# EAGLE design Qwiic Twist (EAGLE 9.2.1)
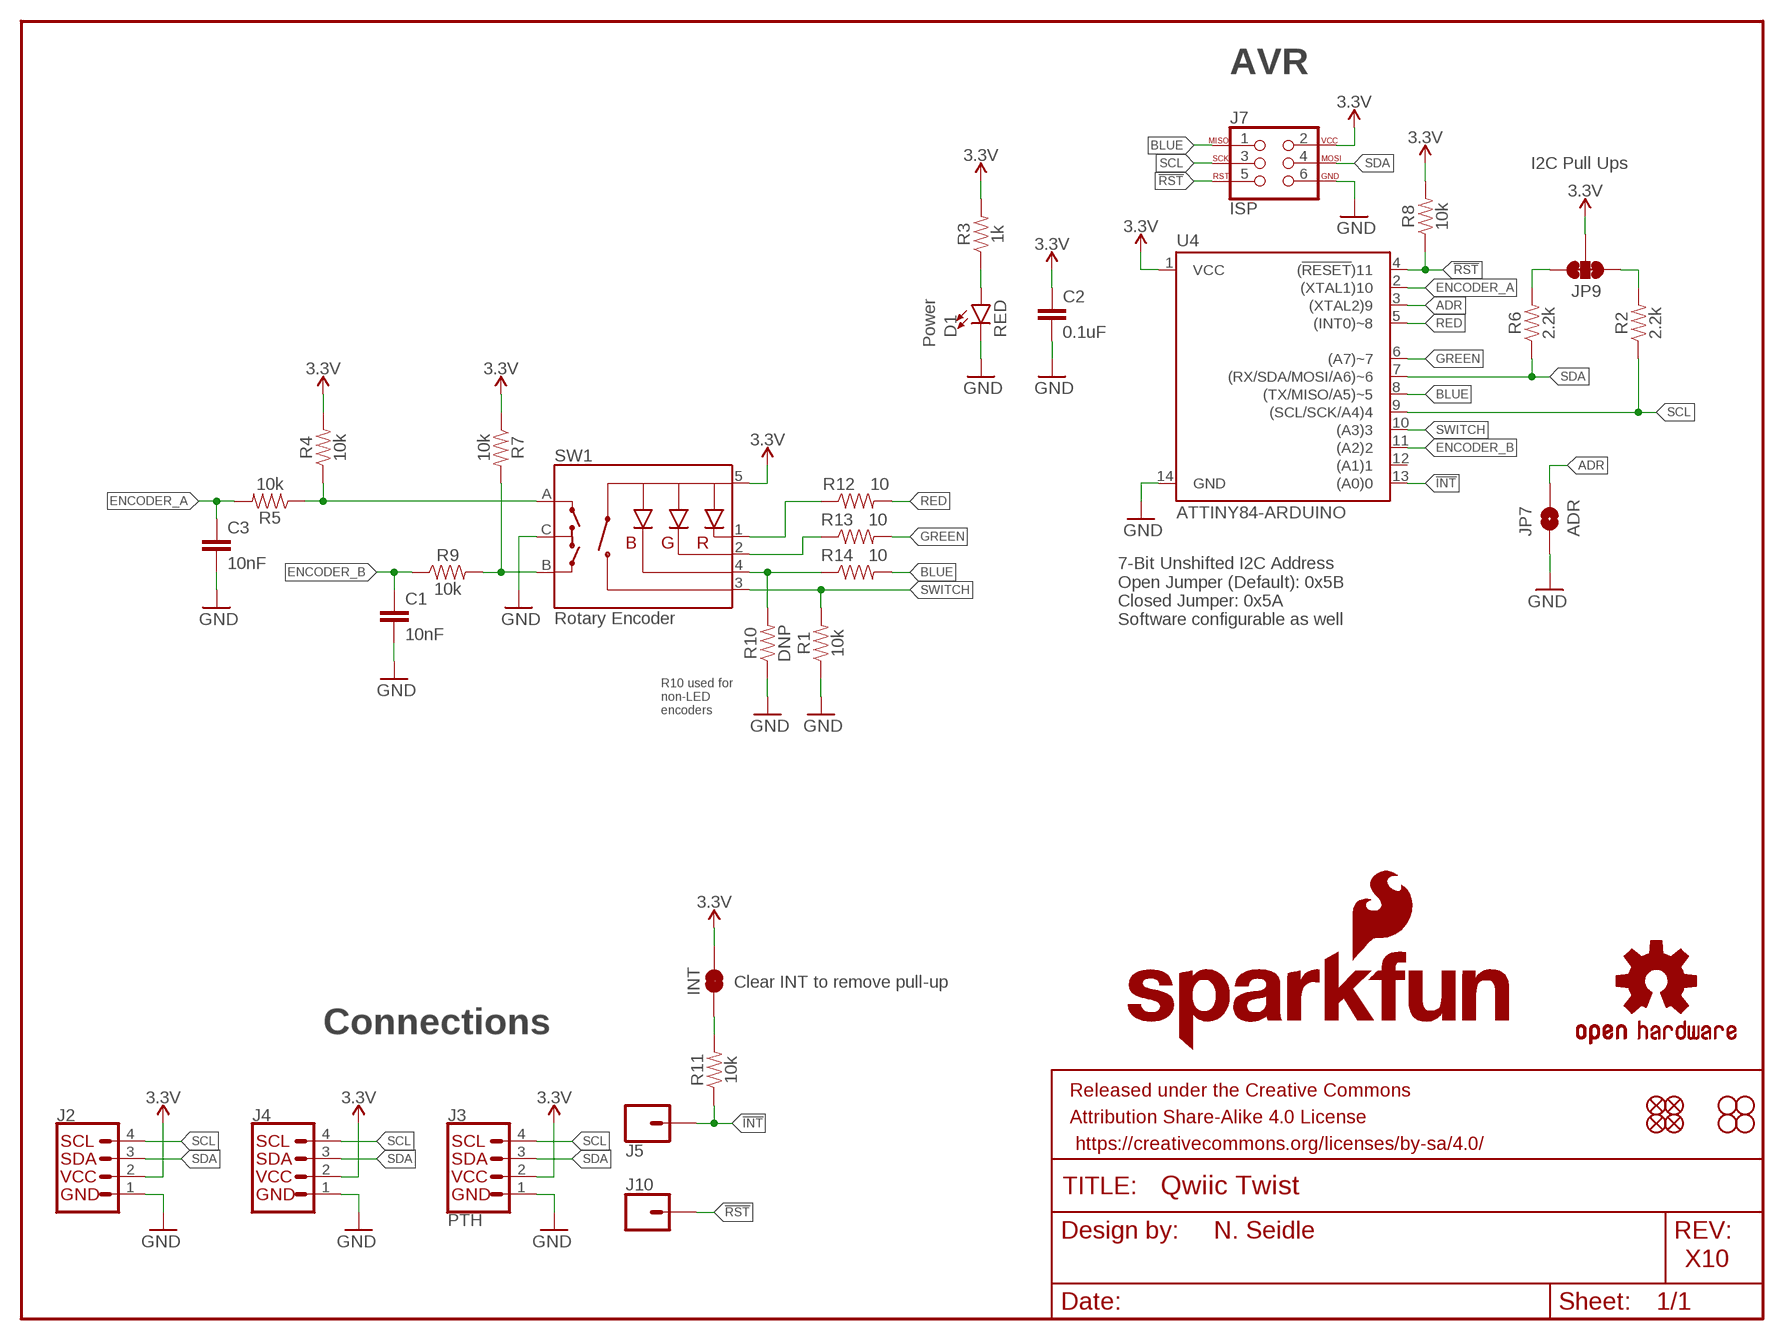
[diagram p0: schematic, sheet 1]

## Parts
C1  10nF  10NF-0603-50V-10%  [0603]
C2  0.1uF  0.1UF-0603-25V-(+80/-20%)  [0603]
C3  10nF  10NF-0603-50V-10%  [0603]
D1  RED  LED-RED0603  [LED-0603]
FRAME1  FRAME-LETTER  [CREATIVE_COMMONS]
INT  JUMPER-SMT_2_NC_TRACE_SILK  [SMT-JUMPER_2_NC_TRACE_SILK]
J2  QWIIC_CONNECTORJS-1MM  [1X04_1MM_RA]
J3  PTH  I2C_STANDARD_NO_SILK  [1X04_NO_SILK]
J4  QWIIC_CONNECTORJS-1MM  [1X04_1MM_RA]
J5  CONN_01PTH_NO_SILK_YES_STOP  [1X01_NO_SILK]
J7  ISP  AVR_SPI_PROG_3X2TESTPOINTS  [2X3_TEST_POINTS]
J10  CONN_01PTH_NO_SILK_YES_STOP  [1X01_NO_SILK]
JP1  FIDUCIALUFIDUCIAL  [MICRO-FIDUCIAL]
JP2  FIDUCIALUFIDUCIAL  [MICRO-FIDUCIAL]
JP3  STAND-OFF  [STAND-OFF]
JP4  STAND-OFF  [STAND-OFF]
JP5  FIDUCIALUFIDUCIAL  [MICRO-FIDUCIAL]
JP6  FIDUCIALUFIDUCIAL  [MICRO-FIDUCIAL]
JP7  ADR  JUMPER-SMT_2_NO_SILK  [SMT-JUMPER_2_NO_SILK]
JP9  JUMPER-SMT_3_2-NC_TRACE_SILK  [SMT-JUMPER_3_2-NC_TRACE_SILK]
JP11  STAND-OFF  [STAND-OFF]
JP13  STAND-OFF  [STAND-OFF]
LOGO1  OSHW-LOGOMINI  [OSHW-LOGO-MINI]
LOGO2  SFE_LOGO_NAME_FLAME.1_INCH  [SFE_LOGO_NAME_FLAME_.1]
LOGO3  SFE_LOGO_FLAME.1EXP  [SFE_LOGO_FLAME_COPPER_EXPOSED_.1]
R1  10k  10KOHM-0603-1/10W-1%  [0603]
R2  2.2k  2.2KOHM-0603-1/10W-1%  [0603]
R3  1k  1KOHM-0603-1/10W-1%  [0603]
R4  10k  10KOHM-0603-1/10W-1%  [0603]
R5  10k  10KOHM-0603-1/10W-1%  [0603]
R6  2.2k  2.2KOHM-0603-1/10W-1%  [0603]
R7  10k  10KOHM-0603-1/10W-1%  [0603]
R8  10k  10KOHM-0603-1/10W-1%  [0603]
R9  10k  10KOHM-0603-1/10W-1%  [0603]
R10  DNP  10KOHM-0603-1/10W-1%  [0603]
R11  10k  10KOHM-0603-1/10W-1%  [0603]
R12  10  10OHM-0603-1/10W-1%  [0603]
R13  10  10OHM-0603-1/10W-1%  [0603]
R14  10  10OHM-0603-1/10W-1%  [0603]
SW1  Rotary Encoder  ENCODER-RGB-SWITCHKIT  [ENCODER_LED_3_KIT]
U4  ATTINY84-ARDUINO  [SO14]

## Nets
3.3V: C2.1 INT.2 J2.2 J3.2(VCC) J4.2 J7.2 JP9.2 R3.2 R4.2 R7.1 R8.2 SW1.5(+) U4.1(VCC)
!INT: J5.1 R11.1 U4.13((A0)0)
!RST: J7.5 J10.1 R8.1 U4.4((!RESET!)11)
A: R4.1 R5.1 SW1.A
ADR: JP7.2 U4.3((XTAL2)9)
B: R7.2 R9.2 SW1.B
BLUE: J7.1 R14.2 U4.8((TX/MISO/A5)~5)
BLUE_RAW: R10.2 R14.1 SW1.4(-B)
ENCODER_A: C3.1 R5.2 U4.2((XTAL1)10)
ENCODER_B: C1.1 R9.1 U4.11((A2)2)
GND: C1.2 C2.2 C3.2 D1.C J2.1 J3.1(GND) J4.1 J7.6 JP7.1 R1.1 R10.1 SW1.C U4.14(GND)
GREEN: R13.2 U4.6((A7)~7)
GREEN_RAW: R13.1 SW1.2(-G)
INT_R: INT.1 R11.2
N$3: D1.A R3.1
RED: R12.2 U4.5((INT0)~8)
RED_RAW: R12.1 SW1.1(-R)
SCL: J2.4 J3.4(SCL) J4.4 J7.3 R2.1 U4.9((SCL/SCK/A4)4)
SCL_PU1: JP9.1 R2.2
SDA: J2.3 J3.3(SDA) J4.3 J7.4 R6.1 U4.7((RX/SDA/MOSI/A6)~6)
SDA_PU1: JP9.3 R6.2
SWITCH: R1.2 SW1.3(SW) U4.10((A3)3)
Unconnected: U4.12((A1)1)

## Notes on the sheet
- AVR
- I2C Pull Ups
- Power
- 7-Bit Unshifted I2C Address
  Open Jumper (Default): 0x5B
  Closed Jumper: 0x5A
  Software configurable as well
- R10 used for 
  non-LED 
  encoders
- Clear INT to remove pull-up
- Connections
- N. Seidle
- X10

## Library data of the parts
C1 C3 = SparkFun-Capacitors:10NF: 0.01uF/10nF/10,000pF ceramic capacitors; PROD_ID: CAP-00867
C2 = SparkFun-Capacitors:0.1UF: 0.1µF ceramic capacitors; PROD_ID: CAP-00810
D1 = SparkFun-LED:LED-RED: Red SMD LED; PROD_ID: DIO-00819
FRAME1 = SparkFun-Aesthetics:FRAME-LETTER: Schematic Frame - Letter
INT = SparkFun-Jumpers:JUMPER-SMT_2_NC_TRACE: Normally closed trace jumper
J2 J4 = SparkFun-Connectors:QWIIC_CONNECTOR: SparkFun I2C Standard Qwiic Connector An SMD 1mm pitch JST connector makes it easy and quick (get it? Qwiic?) to connect I2C devices to each other. The Qwiic system enables fast and solderless connection between popular platforms and various sensors and actuators. We carry 200mm, 100mm, 50mm, and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; PROD_ID: CONN-13694
J3 = SparkX:I2C_STANDARD: SparkFun I2C Standard Pinout Header SparkFun has standardized on a pinout for all I2C based sensor breakouts. This pinout allows I2C boards to be plugged directly into the headers on Arduino Uno compatible boards, and to be daisy chained easily. Example SparkFun Products: SparkFun Atmospheric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
J5 J10 = SparkFun-Connectors:CONN_01: Single connection point. Often used as Generic Header-pin footprint for 0.1 inch spaced/style header connections
J7 = SparkFun-Connectors:AVR_SPI_PROG_3X2: AVR ISP 6 Pin This is the reduced ISP connector for AVR programming. Common on Arduino. This footprint will take up less PCB space and can be used with a 10-pin to 6-pin adapter such as SKU: BOB-08508 **Special note about "TEST_POINT" package. The stop mask is on the top side, so if you want your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
JP1 JP2 JP5 JP6 = SparkFun:FIDUCIAL: Fiducial Alignment Points
JP3 JP4 JP11 JP13 = SparkFun:STAND-OFF: Stand Off
JP7 = SparkFun-Jumpers:JUMPER-SMT_2_NO: Normally open jumper
JP9 = SparkFun-Jumpers:JUMPER-SMT_3_2-NC_TRACE: Normally closed trace jumper (2 of 2 connections) This jumper has a trace between all three pads so they are normally closed (NC). Use a razor knife to open the connection(s). For best results follow the IPC guidelines for cutting traces: Cutout at least 0.063 mm (0.005 in). Remove all loose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
LOGO1 = SparkFun-Aesthetics:OSHW-LOGO: Open-Source Hardware (OSHW) Logo
LOGO2 = SparkFun-Aesthetics:SFE_LOGO_NAME_FLAME: SparkFun Font Logo w/ Flame
LOGO3 = SparkFun-Aesthetics:SFE_LOGO_FLAME: SparkFun Flame Logo
R1 R4 R5 R7-R9 R11 = SparkFun-Resistors:10KOHM: 10kΩ resistor; PROD_ID: RES-00824
R2 R6 = SparkFun-Resistors:2.2KOHM: 2.2kΩ resistor; PROD_ID: RES-08272
R3 = SparkFun-Resistors:1KOHM: 1kΩ resistor; PROD_ID: RES-07856
R10 = SparkFun-Resistors:10KOHM: 10kΩ resistor; PROD_ID: RES-00824; VALUE: 10k
R12-R14 = SparkFun-Resistors:10OHM: 10Ω resistor; PROD_ID: RES-12581
SW1 = SparkFun-Switches:ENCODER-RGB-SWITCH: Illuminated Rotary Encoder w/ RGB LED and select switch Encoders rotate similarly to potentiometers, but they’re different from potentiometers in that an encoder has full rotation without limits. They output gray code so that you can tell how much and in which direction the encoder has been turned.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; PROD_ID: RES-10859; SF_SKU: COM-10982
U4 = SparkFun-IC-Microcontroller:ATTINY84-ARDUINO; PROD_ID: IC-14155

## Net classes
1 3.3V: width 0.152 mm

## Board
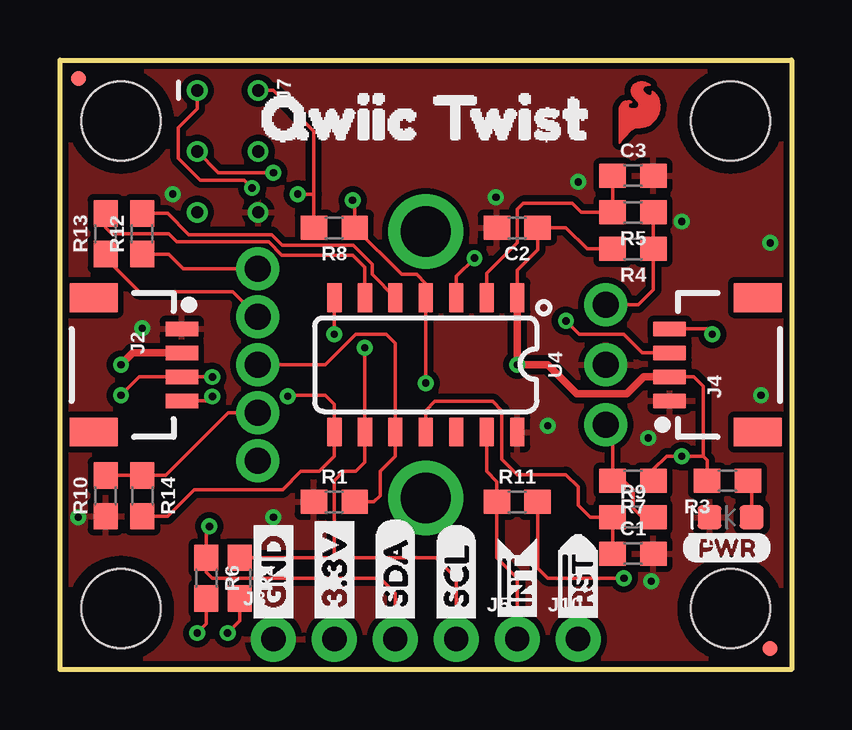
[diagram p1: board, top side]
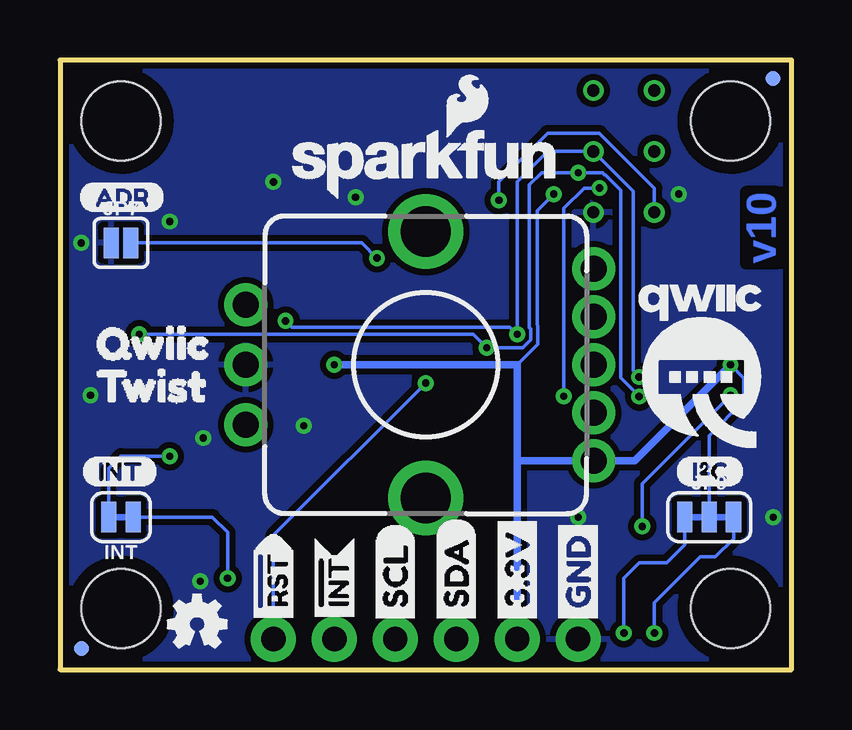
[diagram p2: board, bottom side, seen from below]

Size 30.48 x 25.4 mm. Coordinates in mm from the lower left corner, seen from the top.
Outline: 0,0 0,25.4 30.48,25.4 30.48,0 0,0
Copper layers (1*16): Top 0.035mm / dielectric 1.5mm / Bottom 0.035mm
Design rules "SparkFun-2-layer-PCBWay-LIMIT *": minimum track width 6mil, minimum drill 0.3mm, track to track 6mil, track to pad 6mil, pad to pad 6mil, via to via 6mil, smd to smd 6mil, copper to edge 6mil, drill to drill 6mil, minimum pad ring 7mil, minimum via ring 7mil, stop-mask expansion 4mil, vias tented up to drill 25mil, thermal gap 10mil

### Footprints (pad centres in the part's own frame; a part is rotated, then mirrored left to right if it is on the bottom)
0603 = smd 1.1 x 1: 1 -0.85,0; 2 0.85,0
LED-0603 = smd 1 x 1: A -0.877,0; C 0.877,0
SMT-JUMPER_2_NC_TRACE_SILK = smd 0.635 x 1.27: 1 -0.508,0; 2 0.508,0
1X04_1MM_RA = smd 0.6 x 1.35: 1 -1.5,0; 2 -0.5,0; 3 0.5,0; 4 1.5,0 | smd 1.2 x 2: NC1 2.8,-3.675; NC2 -2.8,-3.675
1X04_NO_SILK = drill 1.016 pad 1.88: 1 0,0; 2 2.54,0; 3 5.08,0; 4 7.62,0
1X01_NO_SILK = drill 1.016 pad 1.88: 1 0,0
2X3_TEST_POINTS = drill 0.508: 1 -2.54,-1.27; 2 -2.54,1.27; 3 0,-1.27; 4 0,1.27; 5 2.54,-1.27; 6 2.54,1.27
MICRO-FIDUCIAL = smd 0.635 x 0.635: 1 0,0
STAND-OFF = hole 3.302: 0,0
SMT-JUMPER_2_NO_SILK = smd 0.635 x 1.27: 1 -0.406,0; 2 0.406,0
SMT-JUMPER_3_2-NC_TRACE_SILK = smd 0.635 x 1.27: 1 -1.016,0; 2 0,0; 3 1.016,0
ENCODER_LED_3_KIT = drill 1.1 pad 1.778: 1 -4,7; 2 -2,7; 3 0,7; 4 2,7; 5 4,7 | drill 1.1 pad 1.8: A -2.5,-7.5; B 2.5,-7.5; C 0,-7.5 | drill 2.1: M1 -5.55,0; M2 5.55,0
SO14 = smd 0.6 x 1.2: 1 -3.175,-2.8; 2 -1.905,-2.8; 3 -0.635,-2.8; 4 0.635,-2.8; 5 1.905,-2.8; 6 3.175,-2.8; 7 4.445,-2.8; 8 4.445,2.8; 9 3.175,2.8; 10 1.905,2.8; 11 0.635,2.8; 12 -0.635,2.8; 13 -1.905,2.8; 14 -3.175,2.8

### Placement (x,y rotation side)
C1  23.88,4.83 0 top
C2  19.05,18.41 180 top
C3  23.88,20.57 0 top
D1  27.94,6.35 180 top
FRAME1  not placed on the board
INT  27.94,6.35 180 bottom
J2  5.08,12.7 270 top
J3  8.89,1.27 0 top
J4  25.4,12.7 90 top
J5  19.05,1.27 0 top
J7  6.99,21.59 270 top
J10  21.59,1.27 0 top
JP1  0.76,24.64 0 bottom
JP2  29.59,0.89 0 top
JP3  2.54,22.86 0 top
JP4  27.94,22.86 0 top
JP5  29.59,0.89 0 bottom
JP6  0.76,24.64 0 top
JP7  27.94,17.78 0 bottom
JP9  3.43,6.35 0 bottom
JP11  2.54,2.54 0 top
JP13  27.94,2.54 0 top
LOGO1  24.77,1.91 0 bottom
LOGO2  15.24,21.08 0 bottom
LOGO3  24.13,23.24 0 top
R1  11.43,6.99 0 top
R2  7.49,3.81 270 top
R3  27.81,7.87 180 top
R4  23.88,17.53 180 top
R5  23.88,19.05 180 top
R6  6.1,3.81 270 top
R7  23.88,7.87 180 top
R8  11.43,18.41 180 top
R9  23.88,6.35 0 top
R10  1.91,7.24 90 top
R11  19.05,6.99 0 top
R12  3.43,18.16 90 top
R13  1.91,18.16 90 top
R14  3.43,7.24 270 top
SW1  15.24,12.7 270 bottom
U4  15.88,12.7 180 top
U$1  [QWIIC1]  30.1,13.59 0 bottom
U$2  [INT0]  29.59,8.26 0 bottom
U$3  [GND1]  8.89,1.65 90 bottom
U$4  [3#3V2]  11.43,1.65 90 bottom
U$5  [SDA8]  13.97,1.65 90 bottom
U$6  [SCL9]  16.51,1.65 90 bottom
U$7  [RST#-[>]  21.59,1.52 90 top
U$8  [I_SUPER2_C-()-03]  4.83,8.26 0 bottom
U$9  [INT#-[<]  19.05,1.52 90 top
U$11  [INT#-[<]  19.05,1.52 90 bottom
U$12  [TWIST2]  30.1,11.81 0 bottom
U$14  [QWIIC_TWIST1]  6.73,22.99 0 top
U$16  [RST#-[>]  21.59,1.52 90 bottom
U$17  [PWR-()-03]  25.91,5.08 0 top
U$18  [ADR-()-03]  29.72,19.68 0 bottom
U$21  [3#3V2]  11.43,1.65 90 top
U$22  [GND1]  8.89,1.65 90 top
U$26  [SCL9]  16.51,1.65 90 top
U$27  [SDA8]  13.97,1.65 90 top
U$47  [QWIIC-LOGO-MEDIUM]  3.81,12.7 0 bottom

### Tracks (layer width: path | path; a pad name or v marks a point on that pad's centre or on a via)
3.3V  (via drill 0.3)
  Top 0.152: U4.1 19.05,16.64 19.9,17.49 C2.1 21.08,18.41 21.97,17.53 R4.2 | J7.2 8.89,24.13 10.58,22.44 10.58,19.81 | R8.2 10.58,19.81 | R7.1 24.73,8.34 25.27,8.89 v25.91,8.89 26.8,8.89 | J4.2 26.41,12.2 26.8,11.81 26.8,8.89 | v9.91,19.81 10.58,19.81 | R3.2 26.96,8.72 26.8,8.89
  Top 0.305: J4.2 24.32,12.2 23.62,11.49 21.52,11.49 20.32,12.7 v19.05,12.7 U4.1 | J2.2 3.04,13.2 v2.54,12.7
  Bottom 0.152: v9.91,19.81 10.6,19.11 10.6,14.37 10.57,14.33 10.57,13.56 11.43,12.7 | INT.2 28.45,8.38 27.94,8.89 v25.91,8.89 | JP9.2 3.43,9.75 1.98,11.2 1.98,12.14 v2.54,12.7
  Bottom 0.305: 8.38,8.7 SW1.5 | SW1.5 6.54,8.7 v2.54,12.7 | J3.2 11.43,8.64 | 11.43,8.64 11.37,8.7 SW1.5 | v19.05,12.7 11.43,12.7 11.43,8.64
!INT
  Top 0.152: J5.1 19.05,3.81 18.2,4.66 R11.1 18.2,7.83 17.78,8.26 U4.13
!RST  (via drill 0.3)
  Top 0.152: v12.19,19.56 12.28,19.47 R8.1 14.23,16.46 14.86,16.46 15.24,16.08 U4.4 v15.24,11.94
  Bottom 0.152: v12.19,19.56 12.19,20.32 10.16,22.35 8,22.35 5.71,20.07 J7.5 | J10.1 21.59,5.59 v15.24,11.94
A
  Top 0.152: R5.1 R4.1 24.73,15.84 24.09,15.2 SW1.A
ADR  (via drill 0.3)
  Top 0.152: U4.3 16.51,16.38 v17.27,17.14
  Bottom 0.152: JP7.2 17.91,17.78 v17.27,17.14
B
  Top 0.152: R9.2 24.26,6.35 23.88,6.73 23.88,7.49 23.5,7.87 R7.2 23.03,9.91 SW1.B
BLUE  (via drill 0.3)
  Top 0.152: v9.49,11.39 9.53,11.43 11.05,11.43 11.43,11.05 U4.8 11.43,8.89 10.79,8.26 10.03,8.26 9.27,7.49 5.59,7.49 4.48,6.39 R14.2 | v8,20.07 7.67,20.4 5.85,20.4 4.93,21.32 4.93,22.58 5.71,23.37 J7.1
  Bottom 0.152: v9.49,11.39 9.49,19.21 8.64,20.07 v8,20.07
BLUE_RAW
  Top 0.152: R10.2 R14.1 4.41,8.09 7.02,10.7 SW1.4
ENCODER_A
  Top 0.152: C3.1 R5.2 21.72,19.05 21.34,19.43 19.3,19.43 19.05,19.18 19.05,17.78 17.78,16.51 U4.2
ENCODER_B
  Top 0.152: C1.1 R9.1 22.1,6.35 21.59,6.86 21.59,7.62 21.08,8.13 19.05,8.13 18.41,8.76 18.41,10.79 18.03,11.18 15.62,11.18 15.24,10.79 U4.11
GND  (via drill 0.3)
  other vias: 0.76,6.35 3.43,14.22 24.51,9.65 24.64,3.68 25.91,18.67 21.59,20.32 29.59,17.78 18.16,19.68 20.32,10.16 8.89,6.35 4.7,19.81 29.21,11.43
  pour Bottom (isolate 0.254, rank 2): 0,0 0,25.4 30.48,25.4 30.48,0
  pour Top (isolate 0.254, rank 2): 0,0 0,25.4 30.48,25.4 30.48,0
GREEN
  Top 0.152: U4.6 12.7,16.76 12.19,17.27 9.25,17.27 8.7,17.82 4.87,17.82 4.52,18.16 2.16,18.16 1.91,18.41 R13.2
GREEN_RAW
  Top 0.152: R13.1 1.91,17.14 3.3,15.75 7.19,15.75 SW1.2
INT_R  (via drill 0.3)
  Top 0.152: R11.2 19.9,4.23 20.32,3.81 v23.5,3.81
  Bottom 0.152: v23.5,3.81 23.5,5.71 24.13,6.35 INT.1
N$3
  Top 0.152: R3.1 28.82,7.72 D1.A
RED
  Top 0.152: U4.5 13.01,16.46 13.01,16.89 12.21,17.69 9.27,17.69 8.83,18.12 5.37,18.12 4.48,19.01 R12.2
RED_RAW
  Top 0.152: SW1.1 5.14,16.7 4.53,17.31 R12.1
SCL  (via drill 0.3)
  Top 0.152: J2.4 6.17,11.2 v6.35,11.38 | J4.4 26.95,14.2 v27.18,13.97 | v12.7,13.41 U4.9 12.7,8.64 12.32,8.26 11.81,8.26 11.43,7.87 11.43,4.66 | R2.1 11.43,4.66 | 11.43,4.66 15.66,4.66 16.51,3.81 J3.4 | v8.89,20.7 6.6,20.7 J7.3
  Bottom 0.152: v27.18,13.97 13.26,13.97 v12.7,13.41 11.2,13.41 10.87,13.74 10.87,14.2 10.92,14.25 10.92,20.19 10.41,20.7 v8.89,20.7 7.87,20.7 7.8,20.62 7.77,20.62 7.12,19.98 7.12,12.15 v6.35,11.38
SCL_PU1  (via drill 0.3)
  Top 0.152: R2.2 7.49,2.03 v6.99,1.52
  Bottom 0.152: JP9.1 4.45,5.21 5.21,4.45 6.35,4.45 6.99,3.81 v6.99,1.52
SDA  (via drill 0.3)
  Top 0.152: v6.35,12.19 v6.34,12.2 J2.3 3.31,12.2 v2.54,11.43 | J4.3 24.27,13.2 23.5,13.97 21.64,13.97 v21.08,14.53 | v11.43,13.97 U4.7 | J3.3 13.97,3.17 13.34,3.81 6.35,3.81 6.1,4.06 R6.1 6.1,5.84 v6.22,5.97
  Bottom 0.152: v6.35,12.19 6.6,12.45 6.6,19.94 J7.4 10.16,21.59 11.43,20.32 v11.43,13.97 11.73,14.28 20.83,14.28 v21.08,14.53 | v6.22,5.97 6.22,7.75 v2.54,11.43
SDA_PU1  (via drill 0.3)
  Top 0.152: R6.2 6.1,1.91 v5.71,1.52
  Bottom 0.152: JP9.3 2.41,5.46 3.17,4.7 3.81,4.7 5.71,2.79 v5.71,1.52
SWITCH
  Top 0.152: R1.2 13.08,6.99 13.34,7.24 13.34,8.26 13.97,8.89 U4.10 13.97,13.59 13.59,13.97 12.32,13.97 11.05,12.7 SW1.3

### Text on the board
Bottom: v10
